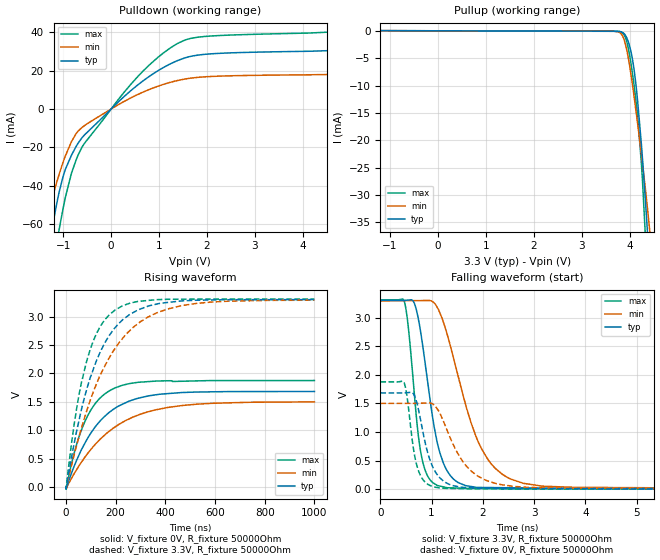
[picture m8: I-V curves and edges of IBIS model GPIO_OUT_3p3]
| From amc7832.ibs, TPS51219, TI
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|   Model
[Model]   GPIO_OUT_3p3
Model_type   Output
Polarity   Non-Inverting
Vmeas = 1.65
Vref = 3.3
Cref = 1pF
Rref = 1000000
|   typ   min   max
C_comp   1pF   1pF   1pF
[Voltage Range]   3.3   3.29   3.31
[Temperature Range]   27   125   -40
[Pullup Reference]   3.3   3.29   3.31
[Pulldown Reference]   -0   -0   -0
[Power Clamp Reference]   3.3   3.29   3.31
[GND Clamp Reference]   -0   -0   -0
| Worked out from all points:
|   slope of the pulldown table from 0 to 0.495 V, typ, clamps not added: 43.8 ohm
|   slope of the pullup table from 0 to 0.495 V, typ, clamps not added: 48 kohm
|   falling waveform, V_fixture 3.3V, R_fixture 50000Ohm: 20-80 % time 349ps typ, 676ps min, 218ps max; typ from 3.3 V to 0.005 V
|   rising waveform, V_fixture 0V, R_fixture 50000Ohm: 20-80 % time 153ns typ, 212ns min, 103ns max; typ from 0.003 V to 1.68 V
|   rising waveform, V_fixture 3.3V, R_fixture 50000Ohm: 20-80 % time 142ns typ, 192ns min, 98.1ns max; typ from 0.005 V to 3.3 V
|   falling waveform, V_fixture 0V, R_fixture 50000Ohm: 20-80 % time 297ps typ, 572ps min, 187ps max; typ from 1.68 V to 0.003 V
[Pulldown]
|   Voltage   I(typ)   I(min)   I(max)
-3.3V     -419.6mA   -290.6mA   -555.1mA
-1.439V   -94.11mA   -67.12mA   -128.5mA
-1.36V    -81.72mA   -59.2mA    -111.5mA
-1.231V   -62.58mA   -46.94mA   -85.89mA
-1.082V   -43.33mA   -34.02mA   -62.77mA
-963.6mV  -32.26mA   -25.2mA    -47.33mA
-825mV    -24.07mA   -16.99mA   -33.41mA
-577.5mV  -14.2mA    -9.112mA   -18.76mA
640.2mV   14.12mA    8.472mA    19.04mA
1.531V    26.54mA    15.54mA    35.8mA
2.363V    29.09mA    17.17mA    38.37mA
6.59V     32.01mA    18.79mA    42.54mA
[Pullup]
|   Voltage   I(typ)   I(min)   I(max)
-3.3V     68.73uA    55.4uA     86.42uA
3.828V    -212.4uA   -632.9uA   -253.6uA
3.887V    -574.2uA   -1.774mA   -813.3uA
3.957V    -1.7mA     -4.362mA   -2.685mA
4.036V    -4.273mA   -8.601mA   -6.576mA
4.095V    -7.469mA   -12.35mA   -10.34mA
4.165V    -12.89mA   -17.02mA   -15.67mA
4.244V    -20.89mA   -22.59mA   -24.39mA
4.343V    -33.19mA   -30.23mA   -40.33mA
4.353V    -34.51mA   -31.04mA   -42.17mA
4.422V    -44.1mA    -36.98mA   -55.74mA
6.59V     -417.6mA   -290.4mA   -550.2mA
[Ramp]
R_load = 50000
|   typ   min   max
dV/dt_r   1.00855/1.53481e-07   0.898303/2.1227e-07   1.12453/1.03121e-07
dV/dt_f   1.97696/3.4851e-10   1.96934/6.74554e-10   1.98335/2.18346e-10
[Falling Waveform]
V_fixture = 3.3V
V_fixture_min = 3.29V
V_fixture_max = 3.31V
R_fixture = 50000Ohm
C_fixture = 0F
|   Time   V(typ)   V(min)   V(max)
0s        3.3V       3.29V      3.31V
474.2ps   3.3V       3.294V     3.259V
641.4ps   3.286V     3.296V     1.89V
761.1ps   2.881V     3.297V     797.7mV
963.8ps   1.604V     3.298V     172.1mV
1.164ns   627.9mV    3.074V     55.87mV
1.427ns   178.9mV    2.293V     23.51mV
1.979ns   31.95mV    699.8mV    14.22mV
2.668ns   25.61mV    141.5mV    10.21mV
1us       5.271mV    7.821mV    4.415mV
[Rising Waveform]
V_fixture = 0V
V_fixture_min = 0V
V_fixture_max = 0V
R_fixture = 50000Ohm
C_fixture = 0F
|   Time   V(typ)   V(min)   V(max)
0s        2.654mV    3.536mV    2.465mV
562.9ps   -17.38mV   3.023mV    -35.74mV
21.08ns   230.8mV    145.2mV    390.3mV
43.17ns   474.9mV    309.1mV    755.3mV
87.41ns   862.1mV    592.7mV    1.257V
134.6ns   1.149V     829.8mV    1.556V
198ns     1.39V      1.06V      1.748V
327.5ns   1.601V     1.322V     1.856V
467.5ns   1.665V     1.437V     1.864V
1us       1.684V     1.501V     1.877V
[Rising Waveform]
V_fixture = 3.3V
V_fixture_min = 3.29V
V_fixture_max = 3.31V
R_fixture = 50000Ohm
C_fixture = 0F
|   Time   V(typ)   V(min)   V(max)
0s        5.271mV    7.821mV    4.415mV
43.17ns   988.5mV    737mV      1.389V
63.71ns   1.391V     1.057V     1.871V
87.41ns   1.78V      1.395V     2.278V
134.6ns   2.345V     1.94V      2.801V
198ns     2.808V     2.443V     3.119V
298.5ns   3.133V     2.908V     3.272V
408.4ns   3.25V      3.134V     3.306V
585.9ns   3.294V     3.257V     3.309V
1us       3.3V       3.29V      3.31V
[Falling Waveform]
|Gnd
V_fixture = 0V
V_fixture_min = 0V
V_fixture_max = 0V
R_fixture = 50000Ohm
C_fixture = 0F
|   Time   V(typ)   V(min)   V(max)
0s        1.684V     1.501V     1.877V
463.8ps   1.683V     1.501V     1.862V
697.5ps   1.557V     1.501V     463.9mV
914.2ps   669.5mV    1.508V     94.31mV
1.076ns   300.6mV    1.449V     35.37mV
1.232ns   143.2mV    1.185V     19.06mV
1.55ns    40.85mV    565.7mV    11.52mV
1.865ns   19.59mV    252.9mV    8.964mV
2.994ns   11.43mV    30.79mV    5.59mV
1us       2.654mV    3.536mV    2.465mV
